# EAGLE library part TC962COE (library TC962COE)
TC962COE, Charge Pump Inverting, -18 to -3V, 16-Pin, SOIC W Source: Datasheet
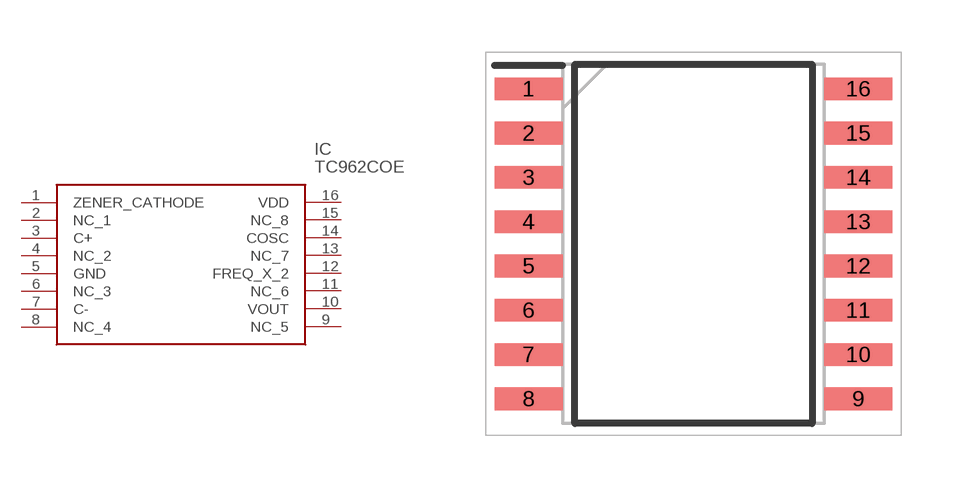
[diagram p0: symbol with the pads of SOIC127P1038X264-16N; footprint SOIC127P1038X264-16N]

Designator prefix IC

## TC962COE (Allied_Number: 70414391; Description: TC962COE, Charge Pump Inverting, -18 to -3V, 16-Pin, SOIC W; Height: 2.64mm; Manufacturer_Name: Microchip; Manufacturer_Part_Number: TC962COE; RS_Part_Number: 6696313P; RS_Price-Stock: http://uk.rs-online.com/web/p/products/6696313P)  [SOIC127P1038X264-16N]
1  ZENER_CATHODE
2  NC_1
3  C+
4  NC_2
5  GND
6  NC_3
7  C-
8  NC_4
9  NC_5
10  VOUT
11  NC_6
12  FREQ_X_2
13  NC_7
14  COSC
15  NC_8
16  VDD

## Footprint SOIC127P1038X264-16N (pad centres in mm)
TC962COE
smd 1.952 x 0.65: 1 -4.724,4.445; 2 -4.724,3.175; 3 -4.724,1.905; 4 -4.724,0.635; 5 -4.724,-0.635; 6 -4.724,-1.905; 7 -4.724,-3.175; 8 -4.724,-4.445; 9 4.724,-4.445; 10 4.724,-3.175; 11 4.724,-1.905; 12 4.724,-0.635; 13 4.724,0.635; 14 4.724,1.905; 15 4.724,3.175; 16 4.724,4.445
